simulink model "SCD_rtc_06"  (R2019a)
settings: Solver=VariableStepAuto  StartTime=0.0  StopTime=10.0  RelTol=1e-3
undefined symbols (not defined in the file or in its folder): algo_cfs1_fp

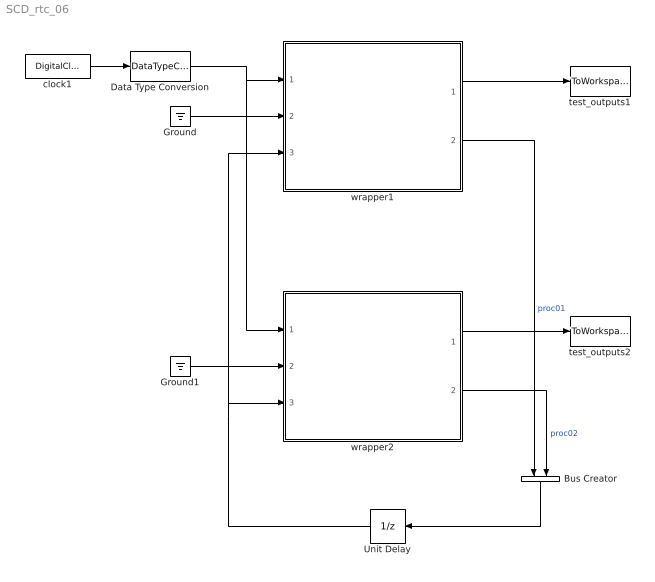
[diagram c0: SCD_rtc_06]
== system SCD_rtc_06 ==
  Bus Creator : BusCreator  Inputs=2
  Data Type Conversion : DataTypeConversion  OutDataTypeStr=single
  Ground : Ground
  Ground1 : Ground
  Unit Delay : UnitDelay  SampleTime=-1  HasFrameUpgradeWarning=on
  clock1 : DigitalClock  SampleTime=algo_cfs1_fp.timing.dt
  test_outputs1 : ToWorkspace  VariableName=cfs1simout  SaveFormat=Timeseries  SampleTime=-1
  test_outputs2 : ToWorkspace  VariableName=cfs2simout  SaveFormat=Timeseries  SampleTime=-1
  wrapper1 : ModelReference  ModelNameDialog=wrapper1.slx  SimulationMode=Normal  ModelReferenceVersion=1.12
  wrapper2 : ModelReference  ModelNameDialog=wrapper2.slx  SimulationMode=Normal  ModelReferenceVersion=1.6
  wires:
  wrapper1/1 -> test_outputs1/1
  wrapper2/1 -> test_outputs2/1
  wrapper1/2 -> Bus Creator/1  "proc01"
  wrapper2/2 -> Bus Creator/2  "proc02"
  Bus Creator/1 -> Unit Delay/1
  Unit Delay/1 -> wrapper2/3, wrapper1/3
  Ground/1 -> wrapper1/2
  clock1/1 -> Data Type Conversion/1
  Data Type Conversion/1 -> wrapper2/1, wrapper1/1
  Ground1/1 -> wrapper2/2
